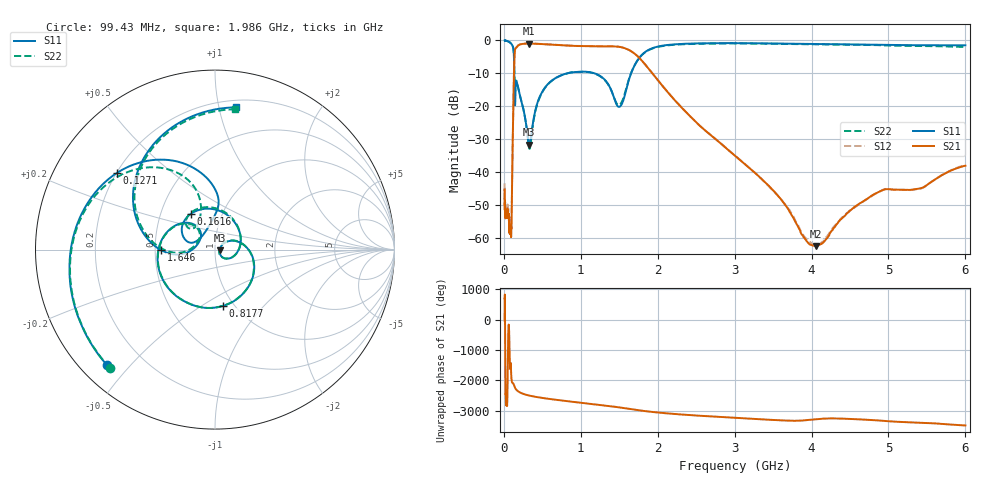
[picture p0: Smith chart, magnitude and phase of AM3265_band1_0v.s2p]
!Agilent Technologies,E8364B,MY43040894,A.07.50.67
!Agilent E8364B: A.07.50.67
!Date: Friday, May 09, 2025 07:13:11
!Correction: S11(Full 2 Port(1,2))
!S21(Full 2 Port(1,2))
!S12(Full 2 Port(1,2))
!S22(Full 2 Port(1,2))
!S2P File: Measurements: S11, S21, S12, S22:Log Frequency Sweep
# Hz S  dB  R 50
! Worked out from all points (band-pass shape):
!   3201 points, 10 MHz to 6 GHz, reference 50 ohm
!   highest |S21| = -0.94 dB at 327.3 MHz (marker M1); lowest = -62.3 dB at 4.055 GHz (marker M2)
!   |S21| within 3 dB of the highest: 140.4 MHz to 1.697 GHz (1.556 GHz wide, 169 % of centre)
!   lowest |S11| = -31.6 dB at 330.6 MHz (marker M3), VSWR 1.05, Z = 52.7 - j0.444 ohm
!   |S11| at or under -10 dB: 135.8 MHz to 815.8 MHz (680 MHz wide, 143 % of centre); 1.185 GHz to 1.653 GHz (468.7 MHz wide, 33 % of centre)
!   |S22| runs from -32.8 to 0.0 dB; largest |S21 - S12| = 0.009
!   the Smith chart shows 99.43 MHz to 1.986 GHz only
!   S11 on the Smith chart (normalised r, x): 99.43 MHz: 0.07, -0.43; 127.1 MHz: 0.20, +0.33; 161.6 MHz: 0.71, +0.30; 817.7 MHz: 0.89, -0.62; 1.646 GHz: 0.54, -0.00; 1.986 GHz: 0.25, +1.12
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1e7  0.01 -11.1  -45.14 -27.7  -43.29 7.5  -0.09 -10.8
2.908064e7  -0.08 -31.9  -52.64 63.0  -52.69 59.2  -0.08 -32.0
8.439949e7  -0.68 -105.2  -58.33 -69.3  -55.72 -159.1  -0.70 -104.9
9.943286e7  -1.09 -133.0  -56.53 -156.3  -54.88 151.0  -1.09 -131.8
1.271496e8  -3.19 141.8  -14.84 34.5  -14.80 34.6  -3.05 148.9
1.616203e8  -12.38 123.9  -2.15 -147.1  -2.12 -147.1  -12.14 115.8
2.44949e8  -19.84 -26.2  -1.03 81.4  -0.99 81.4  -19.85 -26.0
3.27311e8  -31.45 -15.3  -0.94 20.3  -0.90 20.3  -32.48 -19.6
3.305989e8  -31.56 -9.2  -0.94 18.4  -0.90 18.4  -32.72 -13.0
7.123273e8  -10.91 -53.0  -1.38 -132.4  -1.35 -132.4  -10.91 -53.4
8.176802e8  -9.99 -81.6  -1.52 -164.6  -1.49 -164.6  -9.99 -82.3
1.202654e9  -10.16 176.0  -1.80 83.5  -1.77 83.5  -10.24 175.2
1.445482e9  -18.28 130.4  -1.81 7.6  -1.77 7.6  -18.05 133.0
1.646053e9  -10.46 -179.4  -3.14 -65.9  -3.11 -65.9  -10.35 178.2
1.986333e9  -1.93 81.7  -11.58 -177.3  -11.56 -177.2  -2.05 81.8
2.067357e9  -1.55 62.6  -13.91 163.1  -13.89 163.1  -1.67 63.0
2.450248e9  -0.91 -10.3  -23.62 88.5  -23.61 88.4  -1.05 -9.6
2.962692e9  -0.79 -89.3  -34.10 7.8  -34.05 7.6  -0.90 -89.5
3.518433e9  -0.91 -166.6  -45.85 -68.2  -45.92 -68.0  -1.00 -168.4
4.054987e9  -1.07 123.1  -62.33 -44.4  -61.88 129.2  -1.18 120.7
5.002045e9  -1.35 4.2  -45.05 -109.0  -45.02 -108.7  -1.53 4.7
6e9  -1.45 -115.3  -37.94 112.5  -37.76 112.5  -1.96 -111.0
